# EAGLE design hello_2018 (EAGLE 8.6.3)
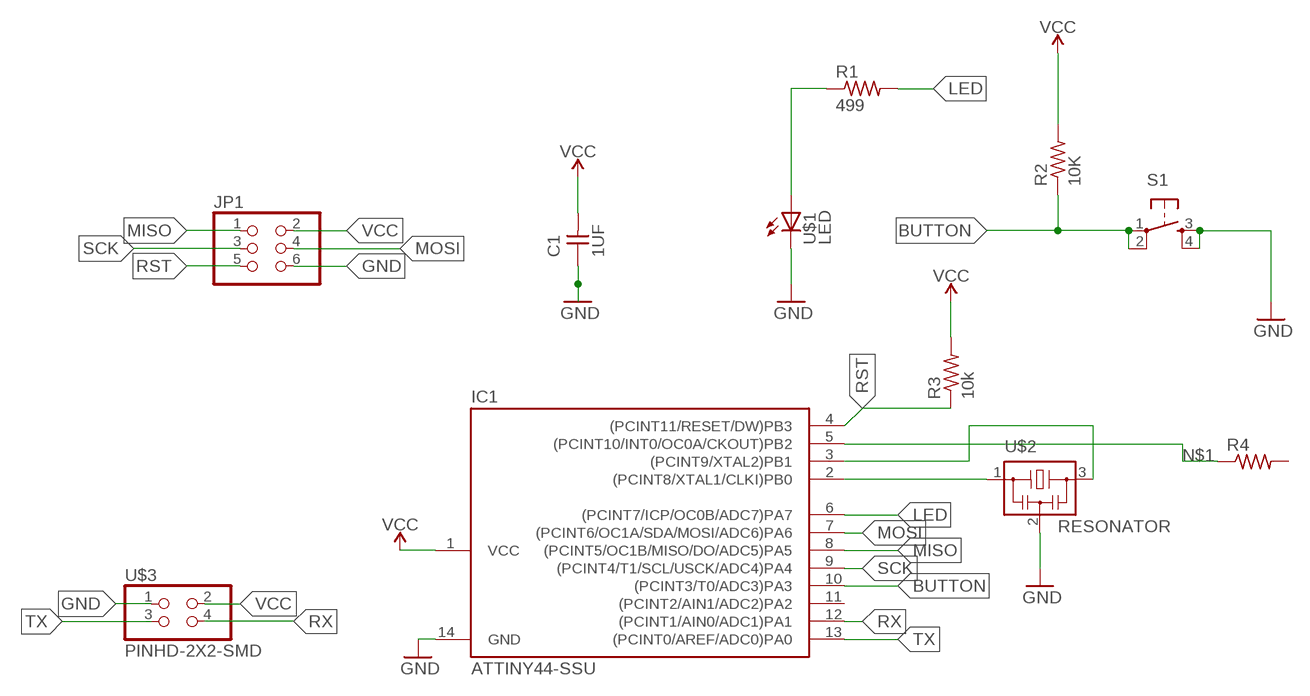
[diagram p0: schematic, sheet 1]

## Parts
C1  1UF  CAP-UNPOLARIZED  [C1206]
IC1  ATTINY44-SSU  [SOIC14]
JP1  PINHD-2X3-SMD  [2X03SMD]
R1  499  RES-US1206  [R1206]
R2  10K  RES-US1206  [R1206]
R3  10k  RES-US1206  [R1206]
R4  RES-US1206  [R1206]
S1  6MM_SWITCH6MM_SWITCH  [6MM_SWITCH]
U$1  LED  [LED1206]
U$2  RESONATOR  [EFOBM]
U$3  PINHD-2X2-SMD  [2X02SMD]

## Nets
BUTTON: IC1.10((PCINT3/T0/ADC3)PA3) R2.1 S1.1(P) S1.2(P1)
GND: C1.1 IC1.14(GND) JP1.6 S1.3(S) S1.4(S1) U$1.2(C) U$2.2 U$3.1
LED: IC1.6((PCINT7/ICP/OC0B/ADC7)PA7) R1.2
MISO: IC1.8((PCINT5/OC1B/MISO/DO/ADC5)PA5) JP1.1
MOSI: IC1.7((PCINT6/OC1A/SDA/MOSI/ADC6)PA6) JP1.4
N$1: IC1.5((PCINT10/INT0/OC0A/CKOUT)PB2) R4.1
N$7: R1.1 U$1.1(A)
N$11: IC1.2((PCINT8/XTAL1/CLKI)PB0) U$2.1
N$12: IC1.3((PCINT9/XTAL2)PB1) U$2.3
RST: IC1.4((PCINT11/RESET/DW)PB3) JP1.5 R3.1
RX: IC1.12((PCINT1/AIN0/ADC1)PA1) U$3.4
SCK: IC1.9((PCINT4/T1/SCL/USCK/ADC4)PA4) JP1.3
TX: IC1.13((PCINT0/AREF/ADC0)PA0) U$3.3
VCC: C1.2 IC1.1(VCC) JP1.2 R2.2 R3.2 U$3.2
Unconnected: IC1.11((PCINT2/AIN1/ADC2)PA2) R4.2

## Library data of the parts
C1 = fab:CAP-UNPOLARIZED
IC1 = fab:ATTINY44
JP1 = fab:PINHD-2X3-SMD: PIN HEADER
R1-R3 = fab:RES-US: Resistor (US Symbol)
R4 = fab2018:RES-US: Resistor (US Symbol)
S1 = fab:6MM_SWITCH: OMRON SWITCH
U$1 = fab:LED: LED
U$2 = fab:RESONATOR
U$3 = fab2018:PINHD-2X2-SMD

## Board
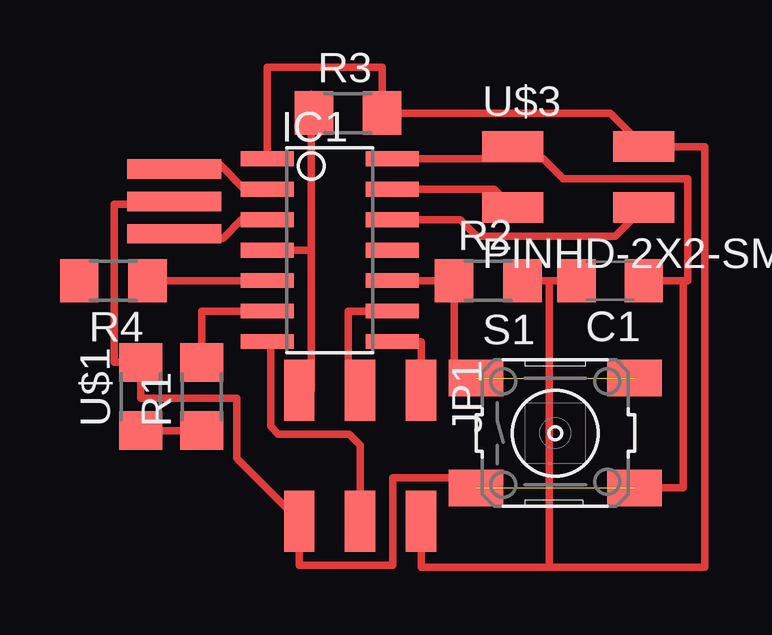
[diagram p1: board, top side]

No outline drawn. Coordinates in mm, seen from the top.
Copper layers (1*16): Top 0.035mm / dielectric 1.5mm / Bottom 0.035mm
Design rules "default *": minimum track width 6mil, minimum drill 0.35mm, track to track 16mil, track to pad 16mil, pad to pad 16mil, via to via 16mil, smd to smd 16mil, copper to edge 40mil, drill to drill 6mil, minimum pad ring 10mil, minimum via ring 8mil, stop-mask expansion 4mil, vias tented up to drill 0mil, thermal gap 10mil

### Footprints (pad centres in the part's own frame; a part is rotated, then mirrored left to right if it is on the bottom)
C1206 = smd 1.6 x 1.8: 1 -1.4,0; 2 1.4,0
SOIC14 = smd 0.61 x 2.21: 1 -3.81,-2.603; 2 -2.54,-2.603; 3 -1.27,-2.603; 4 0,-2.603; 5 1.27,-2.603; 6 2.54,-2.603; 7 3.81,-2.603; 8 3.81,2.603; 9 2.54,2.603; 10 1.27,2.603; 11 0,2.603; 12 -1.27,2.603; 13 -2.54,2.603; 14 -3.81,2.603
2X03SMD = smd 2.54 x 1.27: 1 -2.54,2.54; 2 2.92,2.54; 3 -2.54,0; 4 2.92,0; 5 -2.54,-2.54; 6 2.92,-2.54
R1206 = smd 1.6 x 1.803: 1 -1.422,0; 2 1.422,0
6MM_SWITCH = smd 2.286 x 1.524: 1 -3.302,2.286; 2 3.302,2.286; 3 -3.302,-2.286; 4 3.302,-2.286
LED1206 = smd 1.6 x 1.803: 1 -1.422,0; 2 1.422,0
EFOBM = smd 0.8 x 3.9: 1 -1.35,0; 2 0,0; 3 1.35,0
2X02SMD = smd 2.54 x 1.27: 1 -2.54,1.27; 2 2.92,1.27; 3 -2.54,-1.27; 4 2.92,-1.27

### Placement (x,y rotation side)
C1  33.27,17.78 180 top
IC1  21.59,19.05 270 top
JP1  22.86,10.67 270 top
R1  16.26,12.95 90 top
R2  28.19,17.78 0 top
R3  22.35,24.77 0 top
R4  12.57,17.78 180 top
S1  30.99,11.43 0 top
U$1  13.72,12.95 90 top
U$2  15.11,21.08 270 top
U$3  31.75,22.1 0 top

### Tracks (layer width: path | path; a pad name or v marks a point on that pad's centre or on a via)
BUTTON  (1 unrouted)
  Top 0.305: IC1.10 R2.1 26.77,13.72 S1.1
GND  (1 unrouted)
  Top 0.305: C1.1 36.32,17.78 36.32,9.14 S1.4 | 30.48,22.86 31.32,22.02 36.5,22.02 36.5,17.78 C1.1 | 30.48,22.86 U$3.1 | C1.1 34.67,18.14 | 26.7,9.14 S1.3 27.69,9.58 24.21,9.58 24.21,5.92 20.32,5.92 JP1.6 20.32,7.77 17.72,10.38 17.72,12.89 13.72,12.89 U$1.2 12.6,14.38 12.6,20.95 15.11,20.95 U$2.2 | IC1.14 30.48,22.86
LED
  Top 0.305: 18.06,16.51 IC1.6 16.26,16.51 R1.2
MISO
  Top 0.305: IC1.8 25.4,15.24 JP1.1
MOSI
  Top 0.305: IC1.7 19.13,15.1 19.13,11.71 19.45,11.38 22.4,11.38 22.86,10.92 JP1.4
N$1
  Top 0.305: R4.1 IC1.5
N$7
  Top 0.305: U$1.1 R1.1
N$11
  Top 0.305: IC1.2 18.03,21.59 17.02,22.61 15.11,22.61 U$2.1
N$12
  Top 0.305: IC1.3 17.91,20.32 17.14,19.56 15.11,19.56 U$2.3
RST
  Top 0.305: IC1.4 20.83,19.05 | 20.83,19.05 20.83,13.21 JP1.5 | 20.83,19.05 20.83,25.55 R3.1
RX
  Top 0.305: IC1.12 27.02,20.32 27.71,19.63 33.48,19.63 U$3.4
SCK
  Top 0.305: IC1.9 22.35,16.51 22.35,13.72 22.86,13.72 JP1.3
TX
  Top 0.305: IC1.13 28.45,21.59 U$3.3
VCC
  Top 0.305: JP1.2 25.4,5.84 30.73,5.84 | 30.73,5.84 37.21,5.84 37.21,23.37 U$3.2 33.27,24.77 R3.2 23.77,26.67 18.99,26.67 IC1.1 | R2.2 30.73,17.78 | 30.73,17.78 C1.2 | 30.73,17.78 30.73,5.84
